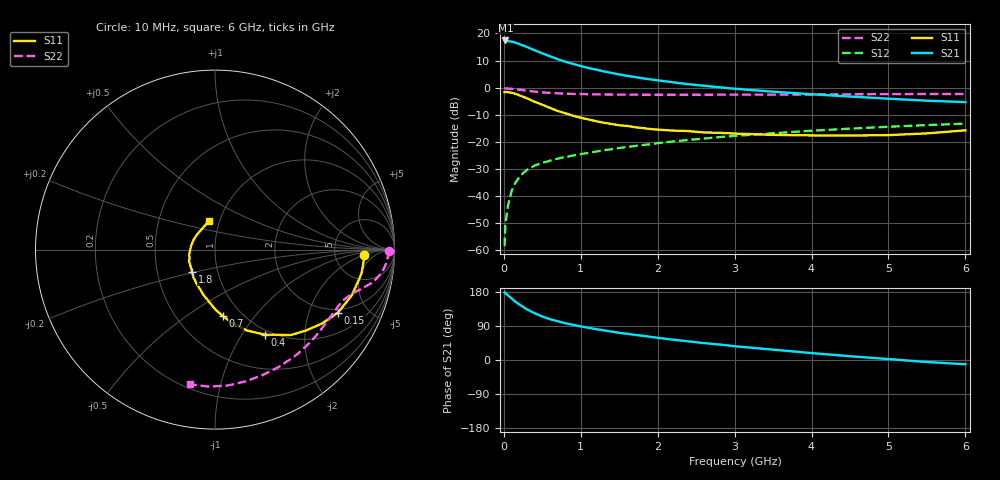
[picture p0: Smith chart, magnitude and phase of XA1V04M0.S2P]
! SIEMENS Discrete & RF Semiconductors
! BFY180
! Si NPN RF Bipolar Junction Transistor in MICRO-X
! VCE = 1 V  IC = 4 mA
! Common Emitter S-Parameters:  May  1997
# GHz  S  MA  R  50
!  f  S11  S21  S12  S22
! GHz  MAG  ANG  MAG  ANG  MAG  ANG  MAG  ANG
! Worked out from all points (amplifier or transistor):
!   36 points, 10 MHz to 6 GHz, reference 50 ohm
!   highest |S21| = 17.4 dB at 20 MHz (marker M1)
!   |S21| within 3 dB of that: start of sweep to 349.7 MHz
!   unconditionally stable (mu >= 1): start of sweep to 11.64 MHz; 576.1 MHz to end of sweep
!   at 250 MHz: K = 0.52, MSG = 23.5 dB, |S12| = -31.5 dB
!   at 1.4 GHz: K = 1.60, MAG = 9.5 dB, |S12| = -22.7 dB
!   at 6 GHz: K = 1.66, MAG = -0.8 dB, |S12| = -13.3 dB
!   S11 on the Smith chart (normalised r, x): 10 MHz: 10, -2; 150 MHz: 1.83, -3.16; 400 MHz: 0.94, -1.27; 700 MHz: 0.82, -0.70; 1.8 GHz: 0.75, -0.20; 6 GHz: 0.89, +0.29
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0.01  0.83 -1.9  7.231 178.4  0.0012 81.3  0.9677 -0.4
0.02  0.8316 -3.7  7.401 176.2  0.003 86.0  0.9687 -1.1
0.05  0.8273 -9.3  7.208 171.2  0.0063 81.3  0.9629 -2.8
0.1  0.804 -18.4  7.054 162.6  0.0124 79.2  0.9523 -5.5
0.15  0.7703 -27.1  6.761 154.2  0.0177 74.0  0.9374 -7.9
0.2  0.7249 -34.6  6.368 146.8  0.0225 69.3  0.917 -9.9
0.3  0.6369 -48.4  5.619 133.6  0.0305 63.2  0.8773 -12.9
0.4  0.5494 -59.6  4.881 123.3  0.0366 58.5  0.8452 -15.0
0.5  0.4845 -68.5  4.279 114.8  0.0413 55.8  0.8178 -16.7
0.6  0.4238 -76.5  3.774 107.6  0.045 54.5  0.8 -18.0
0.7  0.3712 -83.4  3.351 102.4  0.0493 53.0  0.7865 -19.4
0.8  0.3374 -89.1  2.999 97.0  0.0528 52.7  0.7751 -20.6
1  0.2789 -99.4  2.504 88.6  0.0597 52.2  0.7609 -23.3
1.1  0.2593 -104.7  2.303 85.1  0.0627 51.9  0.7553 -24.6
1.4  0.214 -119.3  1.864 74.9  0.0734 51.1  0.7457 -29.1
1.8  0.1803 -135.5  1.491 64.0  0.0874 50.3  0.7405 -35.3
2.2  0.1618 -149.4  1.255 53.7  0.1018 48.0  0.7398 -41.6
3  0.1425 -173.5  0.955 36.4  0.129 43.0  0.7419 -54.0
3.5  0.1349 171.5  0.842 27.3  0.1447 39.8  0.744 -61.6
4.5  0.1309 142.9  0.686 10.0  0.1755 32.1  0.7535 -76.8
5.5  0.1437 114.1  0.575 -5.3  0.2043 24.0  0.764 -92.6
6  0.1635 101.7  0.541 -11.2  0.2175 19.7  0.7638 -100.5
